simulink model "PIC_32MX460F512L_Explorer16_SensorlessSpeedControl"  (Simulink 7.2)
settings: Solver=FixedStepDiscrete  StartTime=0.0  StopTime=10.0  FixedStep=.002  RelTol=1e-3
undefined symbols (not defined in the file or in its folder): bits, Buffer, characters, contain, DiscIntNeverNeededParam, full, is, OC_HW, OCmax, PWM, Receive, Timer3, When
libraries: dsPICdrivers x8, simulink x3

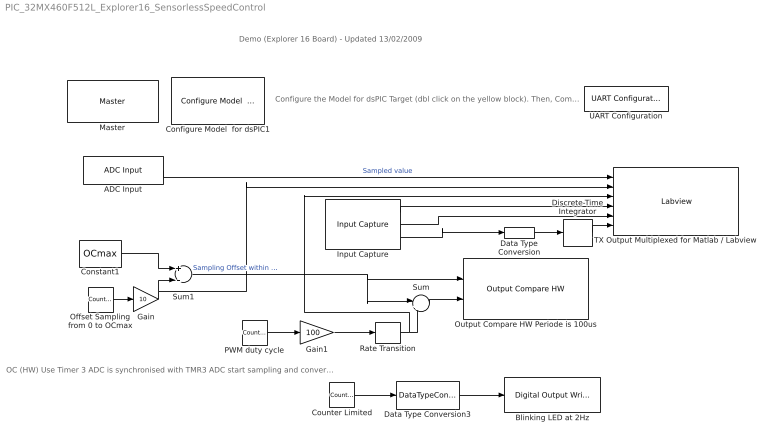
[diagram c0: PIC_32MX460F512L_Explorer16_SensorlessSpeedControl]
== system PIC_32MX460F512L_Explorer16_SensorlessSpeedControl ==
  note: Demo (Explorer 16 Board) - Updated 13/02/2009
  note: Configure the Model for dsPIC Target (dbl click on the yellow block). Then, Compile using the incremental build icon (second icon on right of the simulation mode (Normal))
  note: OC (HW) Use Timer 3 ADC is synchronised with TMR3 ADC start sampling and converting when TMR3 = OCmax (=PR3)
  ADC Input : dsPICdrivers/Peripheral I//O/ADC Input  Tag=dsPIC_ADC  Priority=5  ADC_TYPE=10 bits  ADC_MODE=Continuous sampling & get last channel value  NbrSampleStep=1  VoltRefpopup="AVdd  -  AVss"  OutFormatBitspopup=0000 00dd dddd dddd : Integer  InterruptPriority=6  ANCHANNELS=5  MaxName=ANmax = 1024  Rin=5e6  ADCS=29  SAMC=31  Temperature=25  DMAChannel=0  SampleTime=.002  Status="OK  |  Tsmp=4.844e-006 |  T/Channel=6.719e-006 |  Tall=6.719e-006"  SSRC=Timer3 (OC_HW PWM)
  Blinking LED at 2Hz : dsPICdrivers/Digital I//O/Digital Output Write  Tag=dsPIC_Digital_Output  Priority=5  PORT=A  Pin=[2]  Simultaneous=off  OrderingInOutPopup=None
  Configure Model  for dsPIC1 : dsPICdrivers/Simulink Configuration/Configure Model  for dsPIC
  Constant1 : Constant  Value=OCmax  OutDataTypeMode=uint16  OutDataType=sfix(16)  OutScaling=2^0  OutDataTypeStr=uint16
  Counter Limited : simulink/Sources/Counter Limited  SystemSampleTime=-1  uplimit=1  tsamp=.25
  Data Type Conversion : DataTypeConversion  OutDataTypeMode=uint16  OutDataType=sfix(16)  OutScaling=2^0  OutDataTypeStr=uint16
  Data Type Conversion3 : DataTypeConversion  OutDataTypeMode=boolean  OutDataType=sfix(16)  OutScaling=2^0  OutDataTypeStr=boolean
  Discrete-Time Integrator : DiscreteIntegrator  gainval=500  SampleTime=-1  OutDataTypeMode=uint16  OutDataType=sfix(16)  OutScaling=2^0  OutDataTypeStr=uint16  ICPrevOutput=DiscIntNeverNeededParam  ICPrevScaledInput=DiscIntNeverNeededParam
  Gain : Gain  Gain=10  ParameterDataType=sfix(16)  ParameterScaling=2^0  OutDataTypeMode=uint16  OutDataType=sfix(16)  OutScaling=2^0  OutDataTypeStr=uint16
  Gain1 : Gain  Gain=100  ParameterDataType=sfix(16)  ParameterScaling=2^0  OutDataTypeMode=uint16  OutDataType=sfix(16)  OutScaling=2^0  OutDataTypeStr=uint16
  Input Capture : dsPICdrivers/Peripheral I//O/Input Capture  Tag=dsPIC_PWM_IC  Priority=5  IntPriority=7  Channel=[1 ]  Channel_UP_Down_Periode=[3]  MaxChannel=[0.15]  SafeMarge=[10]  MaxName=' IC1max '  Precision=[15.917]  Timer=[2]  ChangeDetected=[1]  ChangeDetectedPortRef=3  SampleTime=-1  Status=OK
  Master : dsPICdrivers/Master  Tag=dsPIC_MASTER  Priority=1  TimeStepType=Timer1  picType=32MX460F512L  fcy=96000000  Quartz_33f=8e6  PLLActive_33f=on  fcyDesired_33f=96e6  tmr1="[8  23999  0]"  tmr1Info="Time Step : 0.002  ;   Error : 0%  PR1=23999"  tmr2345="[256    8    0    0]"  tmr2345cfg=[-1 -1 -1 -1]  IOautoConf=on  typePort="[ 0   0  10   0   0   0   0   0   0   0   0   0   0   0   0   0   0   0   0   0   0   8   0   0   0   0   0   0   0   0   0   0   0   0   0   0   0   0   0   0   0   0   0   0   0   0   0   0  24   0   0   0   0   0   0   0   6   0   0   0   0   0   0   0   0   0   0   0   0   0   0   0   0   0   0   0   0   0   0   0   0   0   0   0   4   5   0   0   0   0   0   0   0   0   0   0   0   0   0   0 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"  TRIS="[ 65531  65535  65535  65534  65535  65535  65535 ]"  ADPCFG=0  MasterBusyPort=None  MasterOverloadPort=None  FOSC=Quartz (XT - HS)  ClockSwitchMonitor=Both disabled  TempProtection_33f=TEMP_ON  FPBOR=<empty>  PWRT=disable  MCLR=<empty>  PowerSave=off  OverrideFcy=off  NewFcy=1e6  PR2345="[65535  11999  65535  65535]"
  Offset Sampling from 0 to OCmax : simulink/Sources/Counter Limited  SystemSampleTime=-1  uplimit=round(OCmax/10)  tsamp=.002
  Output Compare HW Periode is 100us : dsPICdrivers/Peripheral I//O/Output Compare HW  Tag=dsPIC_OC_HW_out  Priority=5  OC_Mode=PWM Time Set-Reset (glitch possible)  Timer=3  CHANNEL=[1 ]  Channel_UP_Down_Periode=[16]  PeriodeInput=off  MaxChannel=0.001  MaxName=' OCmax '  Precision=[13.5507]  Status=OK  SafeMarge=[0]  PortLetter=[68]  PortNumber=[0]  MaxValues=[11999]  NPORTS=2
  PWM duty cycle : simulink/Sources/Counter Limited  SystemSampleTime=-1  uplimit=round(OCmax/100)  tsamp=.001*round(OCmax/10)*3
  Rate Transition : RateTransition  Integrity=off
  Sum : Sum  Inputs=|++  OutDataType=sfix(16)  OutScaling=2^0
  Sum1 : Sum  Inputs=+-  OutDataType=sfix(16)  OutScaling=2^0
  TX Output Multiplexed for Matlab / Labview : dsPICdrivers/Serial PORT/TX Output Multiplexed for Matlab // Labview  Tag=dsPIC_TX_Multiplexed  Priority=5  UART=2  CleverSpreadingChk=on  CleverSpreading=1  CHANNEL=[0 1 2 3 4 5]  CHANNELBLOCKED=[]  CHANNELBLOCKED_BITEWISE=0  Status=OK
  UART Configuration : dsPICdrivers/Serial PORT/UART Configuration  Tag=dsPIC_config_UART  Priority=2  UART=2  proposed_BAUD=115200  ALT_TX_RX=on  InterruptTxWhen=When Transmit Buffer is empty  TXInterruptPri=1  TxBufferSize=32  TXEN=on  InterruptRxWhen=When Receive Buffer is full (contain 4 characters)  RXInterruptPri=2  RxBufferSize=32  BAUD=115200  UxBRG=51  Info="UxBRG = 51   ||  Real Baud : 115385   ||  % error : 0.16026  ||  max 23.0769 Bytes / Step"  RealBaud=0
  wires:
  Counter Limited/1 -> Data Type Conversion3/1
  ADC Input/1 -> TX Output Multiplexed for Matlab / Labview/1  "Sampled value"
  Sum/1 -> Output Compare HW Periode is 100us/2
  Sum1/1 -> Output Compare HW Periode is 100us/1, Sum/1  "Sampling Offset within PWM"
  Constant1/1 -> Sum1/1
  Offset Sampling from 0 to OCmax/1 -> Gain/1
  Data Type Conversion3/1 -> Blinking LED at 2Hz/1
  PWM duty cycle/1 -> Gain1/1
  Gain/1 -> Sum1/2, TX Output Multiplexed for Matlab / Labview/2
  Gain1/1 -> Rate Transition/1
  Rate Transition/1 -> Sum/2, TX Output Multiplexed for Matlab / Labview/3
  Input Capture/1 -> TX Output Multiplexed for Matlab / Labview/4
  Input Capture/2 -> TX Output Multiplexed for Matlab / Labview/5
  Input Capture/3 -> Data Type Conversion/1
  Discrete-Time Integrator/1 -> TX Output Multiplexed for Matlab / Labview/6
  Data Type Conversion/1 -> Discrete-Time Integrator/1
